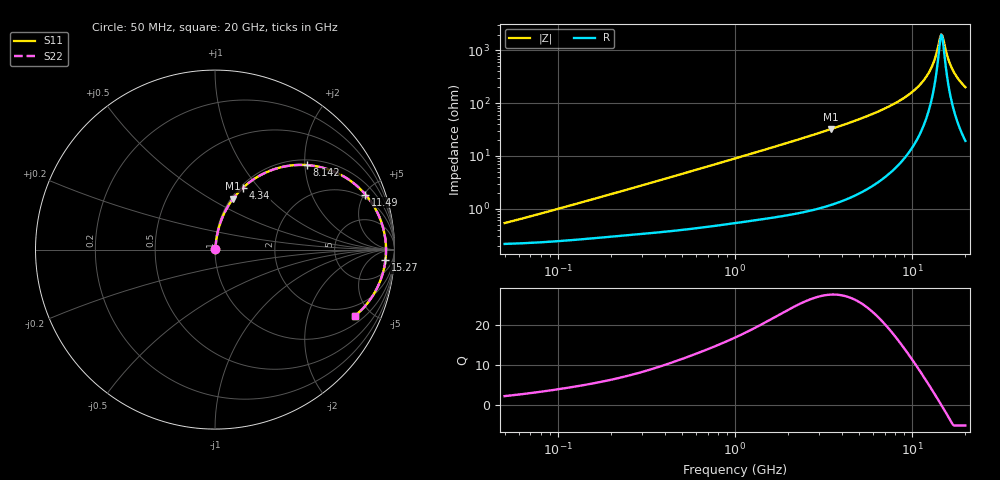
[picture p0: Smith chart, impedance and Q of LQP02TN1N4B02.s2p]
!Murata Part Number: LQP02TN1N4B02
!These Parameters are Measured in Series Mode Connection
!  o--[Z]--o
!Port1  Port2
!  o-------o
!Freq. Start=50[MHz] Stop=20[GHz], 401[Steps]
# Hz S RI R 50
!Freq.(Hz) S11(Real) S11(Imag) S21(Real) S21(Imag) S12(Real) S12(Imag) S22(Real) S22(Imag)
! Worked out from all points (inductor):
!   401 points, 50 MHz to 20 GHz, reference 50 ohm
!   read as one part in series: L = 1.54 nH near 69.52 MHz
!   highest Q = 27.4 at 3.467 GHz (marker M1), where L = 1.47 nH
!   self-resonance near 14.66 GHz
!   S11 on the Smith chart (normalised r, x): 50 MHz: 1.00, +0.01; 4.34 GHz: 1.03, +0.83; 8.142 GHz: 1.12, +2.05; 11.49 GHz: 1.69, +5.10; 15.27 GHz: 16, -20; 20 GHz: 1.39, -4.01
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5e7  0.00217 0.00486  0.9978 -0.00486  0.9978 -0.00486  0.00217 0.00486
1.364002e8  0.00279 0.0129  0.9972 -0.0129  0.9972 -0.0129  0.00279 0.0129
3.721004e8  0.00469 0.0337  0.9953 -0.0337  0.9953 -0.0337  0.00469 0.0337
1e9  0.0131 0.0877  0.9869 -0.0877  0.9869 -0.0877  0.0131 0.0877
2.728004e9  0.0653 0.2289  0.9347 -0.2289  0.9347 -0.2289  0.0653 0.2289
3.466789e9  0.1018 0.2847  0.8982 -0.2847  0.8982 -0.2847  0.1018 0.2847
4.34015e9  0.1561 0.3448  0.8439 -0.3448  0.8439 -0.3448  0.1561 0.3448
5.769027e9  0.27 0.4234  0.73 -0.4234  0.73 -0.4234  0.27 0.4234
7.442007e9  0.4359 0.47  0.5641 -0.47  0.5641 -0.47  0.4359 0.47
8.141811e9  0.5116 0.4709  0.4884 -0.4709  0.4884 -0.4709  0.5116 0.4709
9.892087e9  0.6981 0.4182  0.3019 -0.4182  0.3019 -0.4182  0.6981 0.4182
1.149051e10  0.8384 0.3068  0.1616 -0.3068  0.1616 -0.3068  0.8384 0.3068
1.220001e10  0.8845 0.2432  0.1155 -0.2432  0.1155 -0.2432  0.8845 0.2432
1.295331e10  0.9205 0.1701  0.0795 -0.1701  0.0795 -0.1701  0.9205 0.1701
1.354865e10  0.9393 0.1104  0.0607 -0.1104  0.0607 -0.1104  0.9393 0.1104
1.438523e10  0.952 0.0267  0.048 -0.0267  0.048 -0.0267  0.952 0.0267
1.482269e10  0.9527 -0.0158  0.0473 0.0158  0.0473 0.0158  0.9527 -0.0158
1.527346e10  0.9496 -0.0582  0.0504 0.0582  0.0504 0.0582  0.9496 -0.0582
1.597544e10  0.938 -0.1206  0.062 0.1206  0.062 0.1206  0.938 -0.1206
1.696185e10  0.9103 -0.1991  0.0897 0.1991  0.0897 0.1991  0.9103 -0.1991
1.828096e10  0.8592 -0.2857  0.1408 0.2857  0.1408 0.2857  0.8592 -0.2857
2e10  0.7808 -0.3684  0.2192 0.3684  0.2192 0.3684  0.7808 -0.3684
